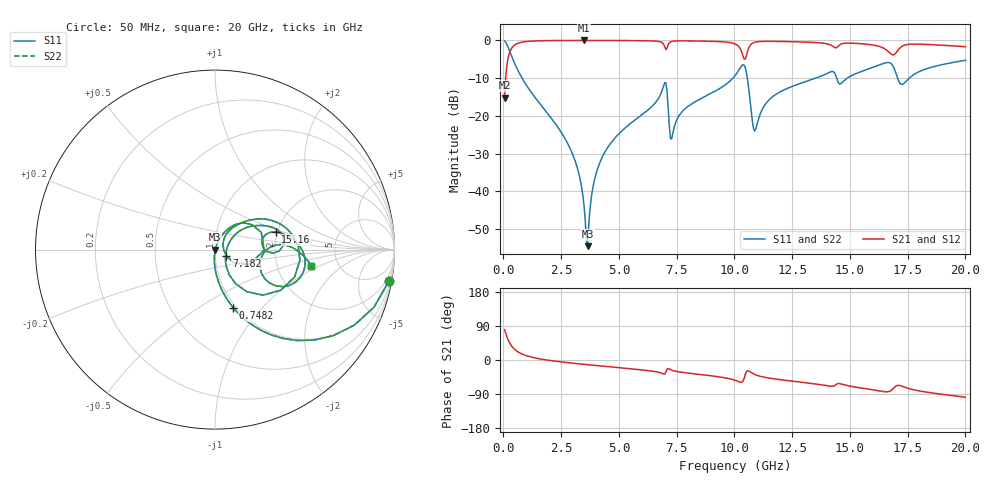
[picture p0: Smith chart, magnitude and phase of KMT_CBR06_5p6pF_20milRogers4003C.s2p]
! Data measured by Modelithics Inc. support@modelithics.com 813-866-6335
! KEMET CBR0603 5.6pF, Pad Width= 0.851mm, Pad Length= 0.64mm, Pad Gap= 0.62mm, 20mil Rogers 4003C substrate Data, January 2022
# hz S ma R 50
! 2 Port Network Data from SP1.SP block
! freq  magS11  angS11  magS21  angS21  magS12  angS12  magS22  angS22
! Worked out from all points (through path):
!   401 points, 50 MHz to 20 GHz, reference 50 ohm
!   highest |S21| = -0.02 dB at 3.491 GHz (marker M1); lowest = -15.2 dB at 50 MHz (marker M2)
!   group delay of S21, straight-line fit = 15.2 ps
!   lowest |S11| = -54.6 dB at 3.641 GHz (marker M3), VSWR 1.00, Z = 50.2 + j0.0405 ohm
!   |S11| at or under -10 dB: 805.3 MHz to 9.936 GHz (9.131 GHz wide, 170 % of centre); 10.56 GHz to 13.52 GHz (2.96 GHz wide, 24.6 % of centre); 17.06 GHz to 17.57 GHz (507.4 MHz wide, 2.93 % of centre)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
!   |S22| runs from -54.6 to -0.1 dB; largest |S21 - S12| = 0
!   S11 on the Smith chart (normalised r, x): 50 MHz: 1, -11; 748.2 MHz: 0.97, -0.71; 7.182 GHz: 1.13, -0.08; 15.16 GHz: 1.96, +0.44; 20 GHz: 3.17, -0.80
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5e7  0.9846 -10.2  0.1747 79.8  0.1747 79.8  0.9846 -10.2
2.99375e8  0.6828 -47.9  0.73 42.0  0.73 42.0  0.6828 -47.9
7.4825e8  0.3396 -72.5  0.9397 17.3  0.9397 17.3  0.3396 -72.5
2.74325e9  0.04523 -94.9  0.9974 -6.7  0.9974 -6.7  0.04523 -94.9
3.391625e9  0.01095 -92.3  0.9982 -10.9  0.9982 -10.9  0.01095 -92.3
3.491375e9  0.006326 -86.3  0.9982 -11.5  0.9982 -11.5  0.006326 -86.3
3.641e9  0.001869 12.5  0.9982 -12.4  0.9982 -12.4  0.001869 12.5
3.94025e9  0.01411 68.6  0.998 -14.2  0.998 -14.2  0.01411 68.6
4.389125e9  0.0329 69.9  0.9974 -16.8  0.9974 -16.8  0.0329 69.9
6.73325e9  0.1748 51.7  0.9677 -32.7  0.9677 -32.7  0.1748 51.7
6.982625e9  0.2752 20.5  0.8247 -37.0  0.8247 -37.0  0.2752 20.5
7.182125e9  0.07267 -28.9  0.9273 -23.9  0.9273 -23.9  0.07267 -28.9
7.33175e9  0.0586 38.4  0.9746 -27.8  0.9746 -27.8  0.0586 38.4
1.0025e10  0.3404 29.4  0.8978 -53.3  0.8978 -53.3  0.3404 29.4
1.0424e10  0.4689 -18.9  0.5639 -48.1  0.5639 -48.1  0.4689 -18.9
1.092275e10  0.06704 6.4  0.9516 -39.3  0.9516 -39.3  0.06704 6.4
1.1621e10  0.1759 37.0  0.9714 -48.9  0.9714 -48.9  0.1759 37.0
1.336662e10  0.3047 26.0  0.9419 -62.1  0.9419 -62.1  0.3047 26.0
1.516212e10  0.3521 16.1  0.916 -70.7  0.916 -70.7  0.3521 16.1
1.670825e10  0.5065 -15.1  0.6914 -82.9  0.6914 -82.9  0.5065 -15.1
1.725688e10  0.2602 -12.0  0.8346 -69.3  0.8346 -69.3  0.2602 -12.0
2e10  0.5445 -9.5  0.8251 -98.1  0.8251 -98.1  0.5445 -9.5
